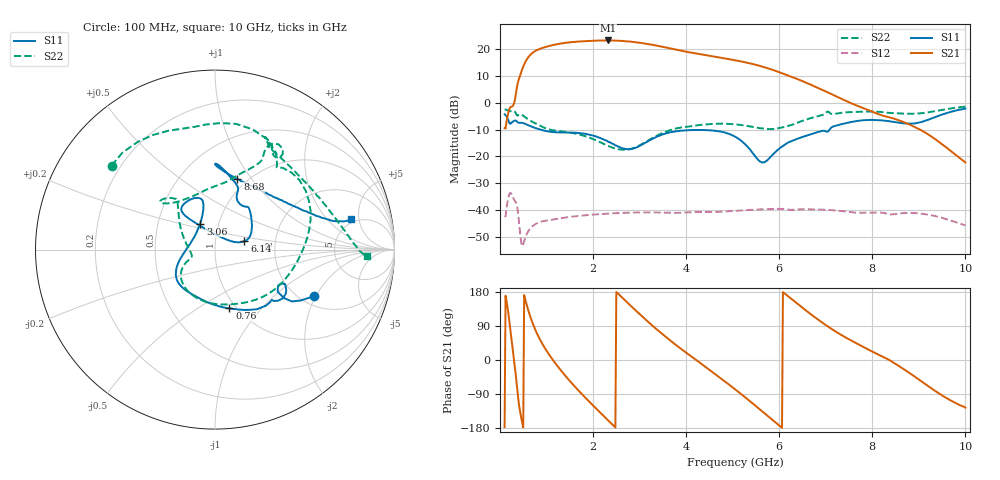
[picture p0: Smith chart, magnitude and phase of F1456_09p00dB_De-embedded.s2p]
! Integrated Device Technology
! Corporate Headquarters
! 6024 Silver Creek Valley Road
! San Jose, CA 95138  USA
! Phone:  1-408-284-8200
! Toll Free:  1-800-223-1366
! Webpage:  http://www.idt.com/
! Timing and RF Division
! 515 Groton Road, Suite 102
! Westford, MA 01886-6024
! Device:  F1456
! Description: 6-bit 0.5 dB Transmit Variable Gain Amplifier
! Frequency:  2100.0 -  2950.00 MHz
! Package:  6x6 mm Thin QFN Plastic Package: 28 pin
! State:  18
! Atten State:  9.0 dB
! Voltage:  +5.00 Volts
! Current:  217.038 mA
! Data:  The device was measured on a the F1455 evaluation board which has
!  individual transmission lines to the RF pins.  Data was collected
!  using a calibrated network analyzer.  The evaluation board was
!  de-embedded using a TRL calibration technique.
!  The reference plane is the edge of the package pin.
!  Pin  1 = CSb
!  Pin  2 = DATA
!  Pin  3 = CLK
!  Pin  4 = RSET
!  Pin  5 = GND
!  Pin  6 = RFIN  = Port 1
!  Pin  7 = GND
!  Pin  8 = NC
!  Pin  9 = NC
!  Pin 10 = NC
!  Pin 11 = NC
!  Pin 12 = NC
!  Pin 13 = NC
!  Pin 14 = /STBY
!  Pin 15 = GND
!  Pin 16 = RFOUT  = Port 2
!  Pin 17 = GND
!  Pin 18 = NC
!  Pin 19 = NC
!  Pin 20 = NC
!  Pin 21 = GND
!  Pin 22 = NC
!  Pin 23 = GND
!  Pin 24 = NC
!  Pin 25 = NC
!  Pin 26 = NC
!  Pin 27 = GND
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# GHz S dB R 50
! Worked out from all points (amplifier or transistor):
!   496 points, 100 MHz to 10 GHz, reference 50 ohm
!   highest |S21| = 23.2 dB at 2.32 GHz (marker M1)
!   |S21| within 3 dB of that: 877.6 MHz to 3.669 GHz (2.791 GHz wide, 123 % of centre)
!   unconditionally stable (mu >= 1): start of sweep to end of sweep
!   at 1.74 GHz: K = 4.09, MAG = 23.5 dB, |S12| = -42.1 dB
!   at 5.06 GHz: K = 6.77, MAG = 16.8 dB, |S12| = -40.3 dB
!   at 10 GHz: K = 142.32, MAG = -12.8 dB, |S12| = -45.7 dB
!   S11 on the Smith chart (normalised r, x): 100 MHz: 2.33, -1.93; 760 MHz: 0.93, -0.69; 3.06 GHz: 0.82, +0.24; 6.14 GHz: 1.38, +0.13; 8.68 GHz: 0.90, +0.85; 10 GHz: 4.59, +3.91
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0.1  -4.31 -25.3  -9.46 -177.2  -42.29 45.7  -2.59 140.9
0.32  -6.65 -32.2  0.98 -18.4  -36.64 -137.2  -3.35 64.7
0.44  -7.46 -43.9  10.57 -141.4  -49.89 142.2  -4.30 39.3
0.58  -8.16 -59.0  16.26 143.0  -48.82 177.3  -5.90 4.5
0.76  -9.46 -76.1  19.33 79.7  -45.30 132.9  -7.67 -27.4
0.98  -10.49 -96.5  20.82 28.5  -44.02 91.8  -9.50 -62.6
1.2  -11.03 -113.5  21.77 -10.3  -43.41 66.2  -10.40 -91.0
1.5  -11.11 -131.5  22.55 -55.3  -42.59 40.4  -11.12 -121.5
1.76  -11.42 -143.2  22.92 -90.0  -42.09 22.4  -12.09 -139.3
2.02  -12.36 -153.4  23.15 -122.5  -41.73 6.7  -13.68 -150.9
2.32  -14.46 -168.3  23.25 -158.9  -41.37 -10.2  -16.09 -158.5
2.66  -17.09 162.3  23.03 160.5  -41.10 -28.2  -17.51 -167.2
3.06  -15.57 119.6  22.24 114.4  -40.91 -48.7  -15.38 165.1
3.4  -12.48 105.8  21.21 77.6  -40.98 -64.9  -12.05 142.0
4.1  -10.19 112.8  18.73 10.5  -40.91 -93.8  -8.77 128.6
5.06  -12.73 130.5  15.84 -78.1  -40.32 -134.4  -8.05 138.8
5.62  -22.21 72.7  13.57 -134.0  -39.77 -163.7  -9.58 124.6
6.14  -15.38 15.9  10.46 173.1  -39.75 165.1  -8.88 87.4
6.7  -11.65 38.8  6.57 118.8  -39.76 134.0  -5.63 64.2
8.36  -6.88 86.7  -5.43 0.4  -41.59 61.3  -3.78 62.4
8.68  -7.69 72.4  -7.26 -24.5  -41.19 52.1  -4.05 52.2
10  -2.18 12.5  -22.28 -125.8  -45.75 -26.5  -1.46 -2.5
